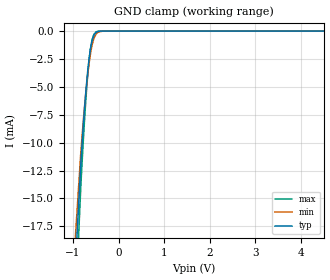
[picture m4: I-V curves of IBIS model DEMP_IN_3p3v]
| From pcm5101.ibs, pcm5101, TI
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|   DEMP_IN_3p3v
[Model]   DEMP_IN_3p3v
Model_type   Input
Vinl = 0.99
Vinh = 2.31
|   typ   min   max
C_comp   0.96423897pF   0.946438018pF   0.978689993pF
[Voltage Range]   3.3   3   3.6
[Temperature Range]   27   105   -25
[Power Clamp Reference]   3.3   3   3.6
[GND Clamp Reference]   -0   -0   -0
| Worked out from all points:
|   GND clamp passes 1 mA (typ) near -0.59 V on its own axis
[GND Clamp]
|   Voltage   I(typ)   I(min)   I(max)
-3.3V     -526.2mA   -489.3mA   -552.6mA
-1.152V   -36.95mA   -31.43mA   -43.61mA
-825mV    -11.69mA   -10.75mA   -13.71mA
-775.5mV  -8.615mA   -8.195mA   -10.02mA
-726mV    -5.891mA   -5.897mA   -6.724mA
-686.4mV  -4.029mA   -4.285mA   -4.478mA
-646.8mV  -2.514mA   -2.918mA   -2.669mA
-617.1mV  -1.636mA   -2.075mA   -1.648mA
-577.5mV  -819uA     -1.212mA   -747.8uA
-478.5mV  -82.94uA   -205.2uA   -52.14uA
-270.6mV  -108.6nA   -1.321uA   -6.009nA
6.6V      0A         0A         0A
[POWER Clamp]
|   Voltage   I(typ)   I(min)   I(max)
-3.3V     0A         0A         0A
0V        0A         0A         0A
6.6V      0A         0A         0A
